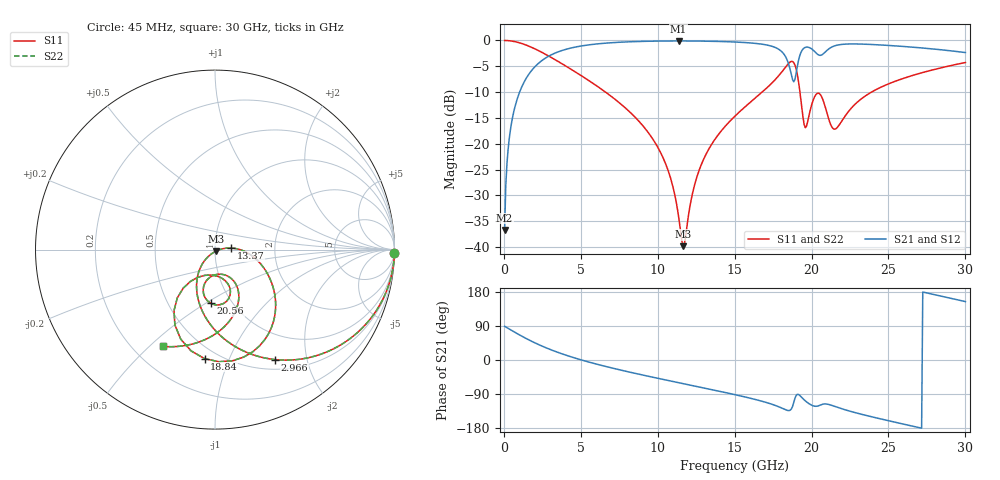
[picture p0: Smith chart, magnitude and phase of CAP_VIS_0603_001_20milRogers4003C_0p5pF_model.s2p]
! S-parameter model data by Modelithics Inc.  support@modelithics.com  813-866-6335  Tampa FL USA
! S-Parameter data specifications:
! Substrate: 20-mil Rogers 4003C, substrate thickness, H=0.508mm, Dielectric constant, Er=3.75
! PCB Mounting Pad Footprint: Pad width, PadW=0.90mm , Pad length, PadL=1.00mm , Pad gap, PadG (edge-to-edge)=1.00mm , Reference planes=3.0mm apart
! Created Wed Nov 18 13:16:27 2015
# hz S ma R 50
! 2 Port Network Data from SP1.SP block
! freq  magS11  angS11  magS21  angS21  magS12  angS12  magS22  angS22
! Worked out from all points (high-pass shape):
!   401 points, 45 MHz to 30 GHz, reference 50 ohm
!   highest |S21| = -0.10 dB at 11.35 GHz (marker M1); lowest = -36.7 dB at 45 MHz (marker M2)
!   |S21| within 3 dB of the highest: 2.88 GHz to 18.3 GHz (15.42 GHz wide, 146 % of centre); 19.22 GHz to end of sweep
!   lowest |S11| = -39.8 dB at 11.65 GHz (marker M3), VSWR 1.02, Z = 50.4 - j0.958 ohm
!   |S11| at or under -10 dB: 6.606 GHz to 16.79 GHz (10.18 GHz wide, 87.1 % of centre); 19.24 GHz to 23.89 GHz (4.649 GHz wide, 21.6 % of centre)
!   |S22| runs from -39.8 to 0.0 dB; largest |S21 - S12| = 0
!   S11 on the Smith chart (normalised r, x): 45 MHz: open; 2.966 GHz: 0.63, -1.50; 13.37 GHz: 1.20, +0.02; 18.84 GHz: 0.42, -0.82; 20.56 GHz: 0.80, -0.53; 30 GHz: 0.32, -0.55
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4.5e7  0.9999 -1.1  0.01463 88.9  0.01463 88.9  0.9999 -1.1
3.4455e8  0.9937 -8.2  0.1114 81.7  0.1114 81.7  0.9937 -8.2
7.93875e8  0.9678 -18.8  0.2508 71.2  0.2508 71.2  0.9678 -18.8
2.965612e9  0.699 -61.3  0.7116 28.5  0.7116 28.5  0.699 -61.3
5.062462e9  0.4528 -89.5  0.8859 -0.2  0.8859 -0.2  0.4528 -89.5
1.007992e10  0.08807 -133.2  0.9864 -48.9  0.9864 -48.9  0.08807 -133.2
1.08288e10  0.04676 -133.7  0.9885 -55.4  0.9885 -55.4  0.04676 -133.7
1.135301e10  0.01989 -120.0  0.989 -59.8  0.989 -59.8  0.01989 -120.0
1.165256e10  0.01021 -68.7  0.9888 -62.4  0.9888 -62.4  0.01021 -68.7
1.247632e10  0.04423 6.3  0.987 -69.4  0.987 -69.4  0.04423 6.3
1.337498e10  0.09183 5.5  0.9826 -77.0  0.9826 -77.0  0.09183 5.5
1.50225e10  0.1855 -6.2  0.9659 -91.5  0.9659 -91.5  0.1855 -6.2
1.8018e10  0.4857 -46.3  0.7901 -126.0  0.7901 -126.0  0.4857 -46.3
1.846732e10  0.5904 -65.0  0.6159 -133.3  0.6159 -133.3  0.5904 -65.0
1.884176e10  0.6102 -95.5  0.3983 -112.3  0.3983 -112.3  0.6102 -95.5
1.914131e10  0.4089 -123.9  0.6303 -90.9  0.6303 -90.9  0.4089 -123.9
1.959064e10  0.1431 -98.3  0.8566 -107.7  0.8566 -107.7  0.1431 -98.3
2.003996e10  0.2477 -69.7  0.8213 -119.9  0.8213 -119.9  0.2477 -69.7
2.056418e10  0.3002 -94.5  0.7171 -119.1  0.7171 -119.1  0.3002 -94.5
2.153771e10  0.1388 -80.8  0.8904 -122.9  0.8904 -122.9  0.1388 -80.8
2.505742e10  0.383 -74.9  0.894 -160.8  0.894 -160.8  0.383 -74.9
3e10  0.6116 -118.1  0.7637 154.1  0.7637 154.1  0.6116 -118.1
